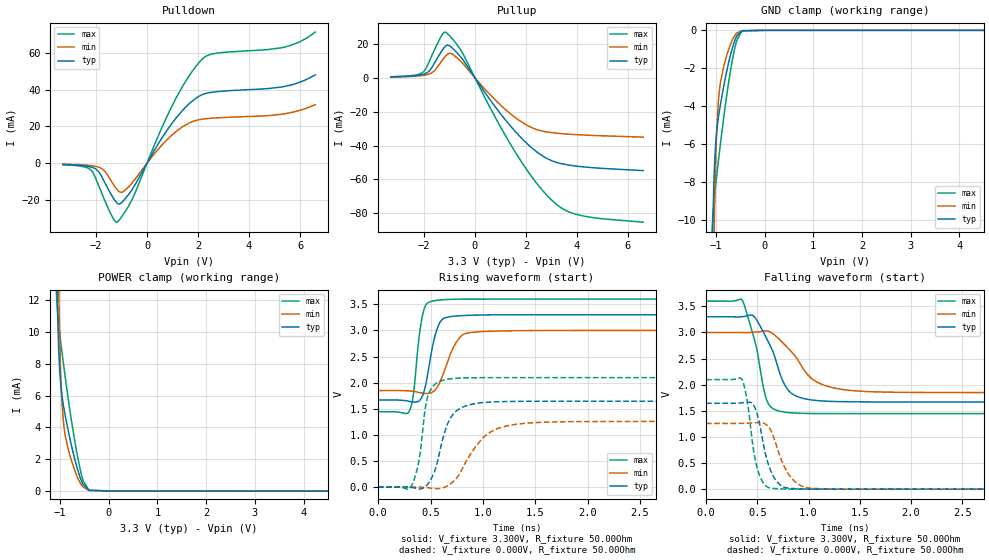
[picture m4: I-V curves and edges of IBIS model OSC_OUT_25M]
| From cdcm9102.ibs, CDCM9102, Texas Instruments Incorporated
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|   OSC_OUT_25M
[Model]   OSC_OUT_25M
Model_type   Output
|Signals   OSC_OUT
Cref = 5pF   |Timing specification test load capacitance value
| variable   typ   min   max
C_comp   0.932pF   0.879pF   1.002pF
[Model Spec]
|Timing spec test load voltage corners 0.45*VCC
Vmeas   3.3V   3.0V   3.6V
Vref   3.3V   3.0V   3.6V
| Junction Temperature (Ambient temp is 15C typ, 85C min,  -40C max)
[Temperature Range]   40.0   100.0   -40.0
[Voltage range]   3.3V   3.0V   3.6V
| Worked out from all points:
|   slope of the pulldown table from 0 to 0.495 V, typ, clamps not added: 41.9 ohm
|   slope of the pullup table from 0 to 0.495 V, typ, clamps not added: 45.5 ohm
|   GND clamp passes 1 mA (typ) near -0.67 V on its own axis
|   POWER clamp passes 1 mA (typ) near -0.60 V on its own axis
|   falling waveform, V_fixture 3.300V, R_fixture 50.00Ohm: 20-80 % time 201ps typ, 292ps min, 140ps max; typ from 3.3 V to 1.67 V
|   rising waveform, V_fixture 3.300V, R_fixture 50.00Ohm: 20-80 % time 96.6ps typ, 140ps min, 69.8ps max; typ from 1.67 V to 3.3 V
|   rising waveform, V_fixture 0.000V, R_fixture 50.00Ohm: 20-80 % time 146ps typ, 261ps min, 85.5ps max; typ from 0 V to 1.65 V
|   falling waveform, V_fixture 0.000V, R_fixture 50.00Ohm: 20-80 % time 121ps typ, 160ps min, 95.2ps max; typ from 1.65 V to 0 V
[Pulldown]
|   Voltage   I(typ)   I(min)   I(max)
-3.3V     -708.7uA   -537.7uA   -850.2uA
-2.181V   -2.149mA   -1.343mA   -3.958mA
-1.718V   -8.902mA   -3.552mA   -18.31mA
-1.307V   -19.38mA   -11.84mA   -30.63mA
-1.174V   -21.79mA   -14.38mA   -32.1mA
-960.9mV  -20.95mA   -15.71mA   -28.49mA
-614.2mV  -14.97mA   -11.24mA   -20.59mA
1.111V    24.14mA    16.93mA    34.73mA
1.628V    32.08mA    21.72mA    47.14mA
2.205V    37.58mA    24.07mA    57.24mA
5.373V    41.77mA    26.88mA    63.23mA
6.598V    48.14mA    31.89mA    71.45mA
[GND Clamp]
|   Voltage   I(typ)   I(min)   I(max)
-3.3V     -1.163A    -1.155A    -1.183A
-1.077V   -12.52mA   -19.9mA    -10.51mA
-1.062V   -10.33mA   -16.3mA    -9.851mA
-1.04V    -8.005mA   -11.81mA   -9.112mA
-1.03V    -7.282mA   -10.19mA   -8.835mA
-1.001V   -5.883mA   -6.686mA   -8.1mA
-975.8mV  -5.179mA   -4.92mA    -7.525mA
-948.5mV  -4.618mA   -3.762mA   -6.913mA
-906.5mV  -3.923mA   -2.782mA   -5.998mA
-666.2mV  -976.2uA   -532.3uA   -1.635mA
-473.3mV  -43.09uA   -22.62uA   -64.41uA
6.598V    0A         0A         0A
[Pullup]
|   Voltage   I(typ)   I(min)   I(max)
-3.3V     597.5uA    498.9uA    664.6uA
-2.035V   2.103mA    1.454mA    3.409mA
-1.649V   7.179mA    3.46mA     14.55mA
-1.278V   16.46mA    10.5mA     25.72mA
-1.139V   18.94mA    13.05mA    26.89mA
-923.8mV  18.08mA    14.28mA    23.69mA
-497.9mV  11.21mA    8.828mA    14.94mA
689.9mV   -14.95mA   -11.42mA   -20.32mA
1.613V    -32.2mA    -23.79mA   -44.62mA
3.007V    -48.91mA   -32.34mA   -72.17mA
4.153V    -52.4mA    -33.66mA   -81.26mA
6.598V    -54.75mA   -34.99mA   -85.23mA
[POWER Clamp]
|   Voltage   I(typ)   I(min)   I(max)
-3.3V     1.174A     1.164A     1.197A
-1.065V   13.49mA    20.95mA    11.94mA
-1.052V   11.58mA    17.86mA    11.36mA
-1.028V   8.951mA    12.81mA    10.5mA
-1.023V   8.562mA    11.95mA    10.35mA
-978.1mV  6.473mA    6.764mA    9.178mA
-933.7mV  5.436mA    4.484mA    8.098mA
-898.8mV  4.822mA    3.6mA      7.283mA
-634mV    1.288mA    790.5uA    2.067mA
-527.6mV  417.3uA    257.8uA    646.5uA
-413.9mV  62.12uA    37.65uA    75.17uA
6.598V    0A         0A         0A
[Ramp]
R_load = 50.00Ohm
|   typ   min   max
dV/dt_r   986.865mV/145.058ps 755.033mV/260.831ps   1.258V/85.276ps
dV/dt_f   978.370mV/200.183ps 690.327mV/291.422ps   1.293V/140.217ps
[Falling Waveform]
V_fixture = 3.300V
V_fixture_min = 3.000V
V_fixture_max = 3.600V
R_fixture = 50.00Ohm
|   Time   V(typ)   V(min)   V(max)
0s        3.3V       3V         3.6V
349.8ps   3.301V     2.998V     3.621V
470.9ps   3.299V     3.004V     2.868V
600.4ps   2.847V     3.028V     1.665V
757.4ps   2.034V     2.785V     1.477V
859.8ps   1.801V     2.569V     1.457V
1.001ns   1.716V     2.17V      1.449V
1.164ns   1.685V     1.982V     1.446V
1.807ns   1.67V      1.856V     1.446V
20ns      1.669V     1.849V     1.446V
[Rising Waveform]
V_fixture = 3.300V
V_fixture_min = 3.000V
V_fixture_max = 3.600V
R_fixture = 50.00Ohm
|   Time   V(typ)   V(min)   V(max)
0s        1.67V      1.849V     1.446V
293.2ps   1.644V     1.843V     1.442V
333.3ps   1.629V     1.835V     1.738V
391.4ps   1.652V     1.813V     2.884V
439.3ps   1.842V     1.794V     3.414V
548.9ps   2.941V     1.873V     3.573V
642.2ps   3.242V     2.282V     3.59V
804.8ps   3.284V     2.912V     3.598V
1.265ns   3.299V     2.993V     3.6V
20ns      3.3V       3V         3.6V
[Rising Waveform]
V_fixture = 0.000V
V_fixture_min = 0.000V
V_fixture_max = 0.000V
R_fixture = 50.00Ohm
|   Time   V(typ)   V(min)   V(max)
0s        -91.58nV   -100.3nV   -77.12nV
317.8ps   -4.312mV   2.353mV    27.17mV
394.3ps   -33.99mV   2.594mV    566mV
454.8ps   18.3mV     -6.13mV    1.575V
537.4ps   300.1mV    -26.25mV   1.961V
659ps     1.194V     22.8mV     2.065V
771.4ps   1.494V     238.6mV    2.088V
1.07ns    1.629V     1.054V     2.096V
1.617ns   1.644V     1.246V     2.097V
20ns      1.645V     1.258V     2.097V
[Falling Waveform]
V_fixture = 0.000V
V_fixture_min = 0.000V
V_fixture_max = 0.000V
R_fixture = 50.00Ohm
|   Time   V(typ)   V(min)   V(max)
0s        1.645V     1.258V     2.097V
348.1ps   1.652V     1.259V     2.106V
396ps     1.662V     1.262V     1.746V
450.4ps   1.641V     1.269V     920.7mV
513.3ps   1.327V     1.274V     310.2mV
602.7ps   506.2mV    1.209V     34.62mV
701ps     121.3mV    742.4mV    7.644mV
888.5ps   8.197mV    109.6mV    640.1uV
1.167ns   642.3uV    6.251mV    4.526uV
20ns      294.8nV    -100.3nV   -68.07uV
